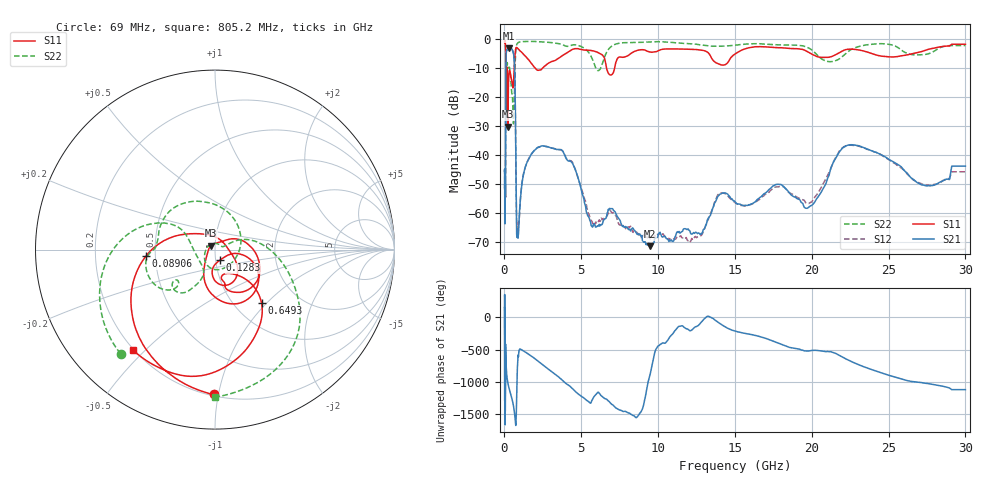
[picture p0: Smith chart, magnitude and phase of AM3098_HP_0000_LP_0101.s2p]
! Date/Time: Thu, Feb 28, 2019 8:30 AM
! Network Analyzer: Agilent Technologies E8364B Rev: A.07.50.67
! Sweep from 0.010 to 30.000 GHz, 1601 Points, Sweep Type: LOG
! Power Supply: 5.022 V, 0.002 A
# Hz S DB R 50
!freq MagS11 AngS11 MagS21 AngS21 MagS12 AngS12 MagS22 AngS22
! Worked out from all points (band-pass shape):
!   1601 points, 10 MHz to 30 GHz, reference 50 ohm
!   highest |S21| = -3.06 dB at 267.8 MHz (marker M1); lowest = -71.3 dB at 9.49 GHz (marker M2)
!   |S21| within 3 dB of the highest: 103.5 MHz to 618.5 MHz (515 MHz wide, 143 % of centre)
!   lowest |S11| = -30.1 dB at 225.9 MHz (marker M3), VSWR 1.06, Z = 47.8 + j2.12 ohm
!   |S11| at or under -10 dB: 175.8 MHz to 631.9 MHz (456.1 MHz wide, 113 % of centre); 2.024 GHz to 2.461 GHz (436.9 MHz wide, 19.5 % of centre); 6.65 GHz to 7.165 GHz (514.5 MHz wide, 7.45 % of centre)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
!   |S22| runs from -29.1 to -0.6 dB; largest |S21 - S12| = 0.0089
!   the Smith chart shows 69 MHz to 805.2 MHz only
!   S11 on the Smith chart (normalised r, x): 69 MHz: 0.21, -0.97; 89.06 MHz: 0.44, -0.04; 128.3 MHz: 1.05, -0.12; 649.3 MHz: 1.32, -0.93; 805.2 MHz: 0.20, -0.46
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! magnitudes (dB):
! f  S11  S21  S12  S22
! 10 MHz  -0.3  -45.5  -45.7  -0.6
! 38.04 MHz  -0.5  -61.5  -61.8  -0.9
! 69 MHz  -1.9  -50.9  -53.5  -2.1
! 89.06 MHz  -8.2  -18.3  -18.2  -9.9
! 97.94 MHz  -24.2  -7.8  -7.8  -17.6
! 112.7 MHz  -13.6  -5.0  -5.0  -10.0
! 128.3 MHz  -23.7  -4.0  -3.9  -11.2
! 144.7 MHz  -13.0  -3.6  -3.5  -10.1
! 185.8 MHz  -11.4  -3.5  -3.5  -8.1
! 225.9 MHz  -30.1  -3.1  -3.1  -9.5
! 267.8 MHz  -14.2  -3.1  -3.0  -9.8
! 550.5 MHz  -16.7  -4.1  -4.1  -24.7
! 649.3 MHz  -8.1  -8.4  -8.4  -18.4
! 805.2 MHz  -2.8  -67.7  -64.8  -1.7
! 2.084 GHz  -10.4  -37.6  -37.6  -0.7
! 3.742 GHz  -5.7  -38.2  -38.3  -1.7
! 5.754 GHz  -3.9  -64.6  -63.7  -7.2
! 7.926 GHz  -5.9  -64.8  -65.6  -1.1
! 9.49 GHz  -4.3  -71.3  -68.8  -0.9
! 19.9 GHz  -4.7  -57.5  -56.3  -3.2
! 22.67 GHz  -3.4  -36.4  -36.5  -3.2
! 30 GHz  -1.7  -43.7  -45.7  -2.1
